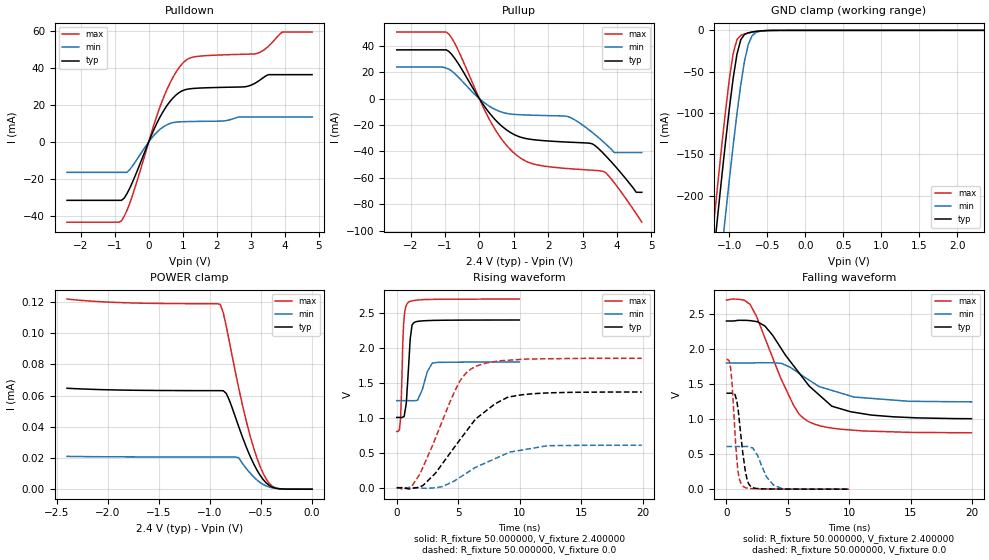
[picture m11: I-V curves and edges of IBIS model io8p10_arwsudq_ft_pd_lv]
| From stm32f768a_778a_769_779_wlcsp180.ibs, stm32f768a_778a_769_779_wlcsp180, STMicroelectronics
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|   Model io8p10_arwsudq_ft_pd_lv
[Model]  io8p10_arwsudq_ft_pd_lv
Model_type I/O
Polarity   Non-Inverting
Enable   Active-Low
Vinl =   0.720000V
Vinh =   1.680000V
Vmeas =  1.200000V
Cref =   40.000000pF
Rref =   100.000000M
Vref =   0.0V
C_comp   2.828000pF   2.774700pF   2.917100pF
[Temperature Range]   25.000000   0.125000k   -40.000000
[Pullup Reference]   2.400000V   1.800000V   2.700000V
[Pulldown Reference]   0.0V   0.0V   0.0V
[POWER Clamp Reference]   2.400000V   1.800000V   2.700000V
[GND Clamp Reference]   0.0V   0.0V   0.0V
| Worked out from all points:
|   slope of the pulldown table from 0 to 0.36 V, typ, clamps not added: 25 ohm
|   slope of the pullup table from 0 to 0.36 V, typ, clamps not added: 27.7 ohm
|   GND clamp passes 1 mA (typ) near -0.62 V on its own axis
|   rising waveform, R_fixture 50.000000, V_fixture 2.400000: 20-80 % time 291ps typ, 618ps min, 206ps max; typ from 1 V to 2.4 V
|   rising waveform, R_fixture 50.000000, V_fixture 0.0: 20-80 % time 3.81ns typ, 3.99ns min, 2.67ns max; typ from 0 V to 1.37 V
|   falling waveform, R_fixture 50.000000, V_fixture 2.400000: 20-80 % time 3.9ns typ, 3.97ns min, 2.74ns max; typ from 2.4 V to 1 V
|   falling waveform, R_fixture 50.000000, V_fixture 0.0: 20-80 % time 547ps typ, 1.01ns min, 409ps max; typ from 1.37 V to 0 V
[Pulldown]
|Voltage   I(typ)   I(min)   I(max)
-2.4V     -31.67mA   -16.51mA   -43.52mA
-800mV    -31.67mA   -16.51mA   -42.86mA
-480mV    -21.98mA   -13.17mA   -29.21mA
80mV      3.63mA     1.966mA    5.012mA
480mV     18.15mA    8.738mA    26.02mA
800mV     25.38mA    10.72mA    37.77mA
1.12V     28.53mA    11.02mA    44.6mA
2.8V      29.84mA    13.49mA    47.53mA
3.2V      32.65mA    13.49mA    48.03mA
3.52V     36.46mA    13.49mA    51.84mA
3.92V     36.46mA    13.49mA    59.54mA
4.8V      36.46mA    13.49mA    59.54mA
[Pullup]
|Voltage   I(typ)   I(min)   I(max)
-2.4V     36.92mA    24.04mA    50.37mA
-960mV    36.92mA    23.06mA    50.37mA
-640mV    27.65mA    17.04mA    37.98mA
320mV     -11.75mA   -6.207mA   -17.08mA
960mV     -26.47mA   -11.82mA   -40.02mA
1.52V     -30.88mA   -12.51mA   -49.05mA
2.56V     -32.88mA   -13.49mA   -52.9mA
3.28V     -34.2mA    -25.52mA   -54.18mA
3.6V      -41.32mA   -32.62mA   -54.99mA
3.92V     -50.34mA   -40.8mA    -63.66mA
4.56V     -70.9mA    -40.8mA    -87.12mA
4.72V     -70.9mA    -40.8mA    -93.5mA
[GND_clamp]
|Voltage   I(typ)   I(min)   I(max)
-2.4V     -1.425A    -1.508A    -1.394A
-1.25V    -311.8mA   -402mA     -274.5mA
-1.2V     -266mA     -356.2mA   -228.4mA
-1.15V    -220.9mA   -310.9mA   -183.1mA
-1.1V     -176.9mA   -266.3mA   -139mA
-1.05V    -134.3mA   -222.6mA   -97.01mA
-950mV    -57.82mA   -139.1mA   -27.87mA
-900mV    -28.73mA   -100.5mA   -11.05mA
-850mV    -11.3mA    -65.69mA   -6.068mA
-750mV    -2.863mA   -16.61mA   -3.194mA
-600mV    -761.3uA   -1.176mA   -752.1uA
2.35V     58.09uA    37.92uA    67.25uA
[POWER_clamp]
|Voltage   I(typ)   I(min)   I(max)
-2.4V     64.71uA    21.03uA    121.9uA
-1.86V    63.55uA    20.74uA    119.6uA
-900mV    63.18uA    20.63uA    118.5uA
-870mV    63.14uA    20.63uA    113.2uA
-840mV    61.36uA    20.62uA    104.3uA
-720mV    40.37uA    20.18uA    65.28uA
-630mV    24.69uA    12.08uA    39.85uA
-540mV    12.26uA    5.907uA    20uA
-480mV    6.236uA    3.061uA    10.23uA
-420mV    2.4uA      1.365uA    3.726uA
-360mV    667.9nA    564nA      839.6nA
0V        0A         0A         0A
[Ramp]
| variable   typ   min   max
dV/dt_r  0.82158/3.80773n   0.36533/3.99238n   1.11053/2.67088n
dV/dt_f  0.83376/3.90093n   0.33300/4.02985n   1.13617/2.74567n
R_load = 50.000000
[Rising Waveform]
R_fixture= 50.000000
V_fixture= 2.400000
V_fixture_min= 1.800000
V_fixture_max= 2.700000
|time   V(typ)   V(min)   V(max)
0s        1.005V     1.245V     804.1mV
220.2ps   1.005V     1.245V     829.8mV
300.3ps   1.005V     1.245V     974.7mV
560.6ps   1.015V     1.246V     2.333V
780.8ps   1.217V     1.246V     2.61V
880.9ps   1.497V     1.246V     2.641V
1.101ns   2.133V     1.245V     2.666V
1.461ns   2.368V     1.245V     2.679V
2.903ns   2.393V     1.782V     2.694V
9.97ns    2.399V     1.799V     2.698V
[Rising Waveform]
R_fixture= 50.000000
V_fixture= 0.0
V_fixture_min= 0.0
V_fixture_max= 0.0
|time   V(typ)   V(min)   V(max)
0s        171.1uV    66.52uV    601.9uV
1.241ns   -9.648mV   180.7uV    26.68mV
1.882ns   15.56mV    -3.26mV    194.6mV
3.163ns   210.3mV    84.68uV    714.8mV
5.005ns   653.8mV    132.4mV    1.483V
6.286ns   953.6mV    278.3mV    1.722V
8.008ns   1.201V     416.4mV    1.805V
9.73ns    1.316V     525.2mV    1.831V
12.29ns   1.356V     601.4mV    1.844V
19.94ns   1.369V     608.4mV    1.85V
[Falling Waveform]
R_fixture= 50.000000
V_fixture= 2.400000
V_fixture_min= 1.800000
V_fixture_max= 2.700000
|time   V(typ)   V(min)   V(max)
0s        2.399V     1.799V     2.698V
1.441ns   2.408V     1.799V     2.696V
1.922ns   2.404V     1.8V       2.637V
3.123ns   2.329V     1.804V     2.16V
4.484ns   1.998V     1.793V     1.558V
5.445ns   1.765V     1.708V     1.202V
6.607ns   1.5V       1.569V     971.5mV
8.569ns   1.185V     1.409V     872.4mV
10.09ns   1.105V     1.329V     844.6mV
19.94ns   1.005V     1.245V     804.1mV
[Falling Waveform]
R_fixture= 50.000000
V_fixture= 0.0
V_fixture_min= 0.0
V_fixture_max= 0.0
|time   V(typ)   V(min)   V(max)
0s        1.369V     608.4mV    1.85V
340.3ps   1.369V     608.4mV    1.728V
440.4ps   1.369V     608.4mV    1.541V
840.8ps   1.26V      608.2mV    436mV
1.041ns   988.8mV    607.9mV    154.5mV
1.321ns   529.6mV    608.1mV    47.07mV
1.702ns   124.6mV    608.9mV    14.73mV
2.162ns   21.14mV    583mV      6.302mV
3.844ns   2.254mV    56.27mV    1.891mV
9.97ns    171.1uV    66.52uV    601.9uV
